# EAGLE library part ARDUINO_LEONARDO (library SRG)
Arduino Leonardo I2C Pins: D2, D3 PWM Pins: D3, D5, D5, D11, D13 Interrup Pint: D2, D3 http://arduino.cc/en/Main/arduinoBoardLeonardo
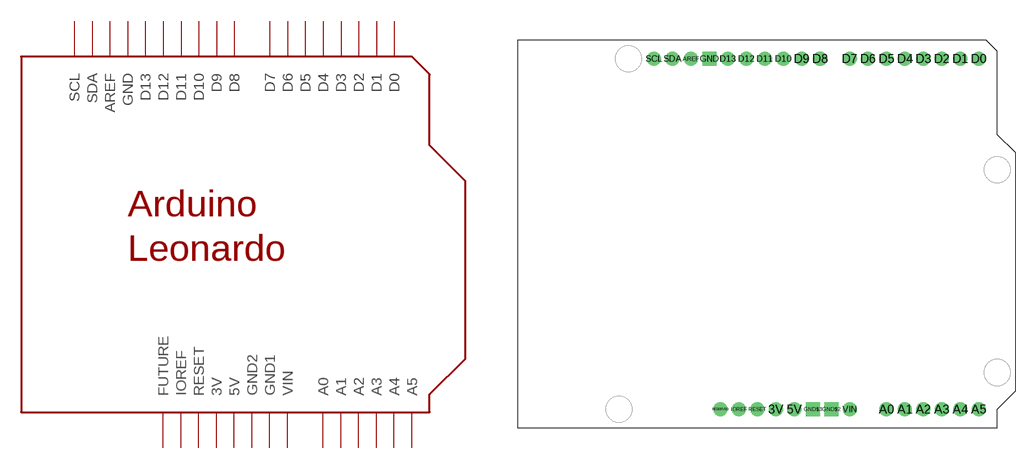
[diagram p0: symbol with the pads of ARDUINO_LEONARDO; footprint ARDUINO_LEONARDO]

Designator prefix -

## ARDUINO_LEONARDO  [ARDUINO_LEONARDO]
3V  3V  pwr
5V  5V  pwr
A0  A0
A1  A1
A2  A2
A3  A3
A4  A4
A5  A5
AREF  AREF
D0  D0
D1  D1
D2  D2
D3  D3
D4  D4
D5  D5
D6  D6
D7  D7
D8  D8
D9  D9
D10  D10
D11  D11
D12  D12
D13  D13
GND  GND  pwr
GND$2  GND2  pwr
GND$3  GND1  pwr
IOREF  IOREF
RESERVED  FUTURE
RESET  RESET
SCL  SCL
SDA  SDA
VIN  VIN  pwr

## Footprint ARDUINO_LEONARDO (pad centres in mm)
Arduino Leonardo pinout
drill 1 pad 1.93: 3V 1.27,-24.13; 5V 3.81,-24.13; A0 16.51,-24.13; A1 19.05,-24.13; A2 21.59,-24.13; A3 24.13,-24.13; A4 26.67,-24.13; A5 29.21,-24.13; AREF -10.414,24.13; D0 29.21,24.13; D1 26.67,24.13; D2 24.13,24.13; D3 21.59,24.13; D4 19.05,24.13; D5 16.51,24.13; D6 13.97,24.13; D7 11.43,24.13; D8 7.366,24.13; D9 4.826,24.13; D10 2.286,24.13; D11 -0.254,24.13; D12 -2.794,24.13; D13 -5.334,24.13; IOREF -3.81,-24.13; RESERVED -6.35,-24.13; RESET -1.27,-24.13; SCL -15.494,24.13; SDA -12.954,24.13; VIN 11.43,-24.13
drill 1 pad 1.93 square: GND -7.874,24.13; GND$2 8.89,-24.13; GND$3 6.35,-24.13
